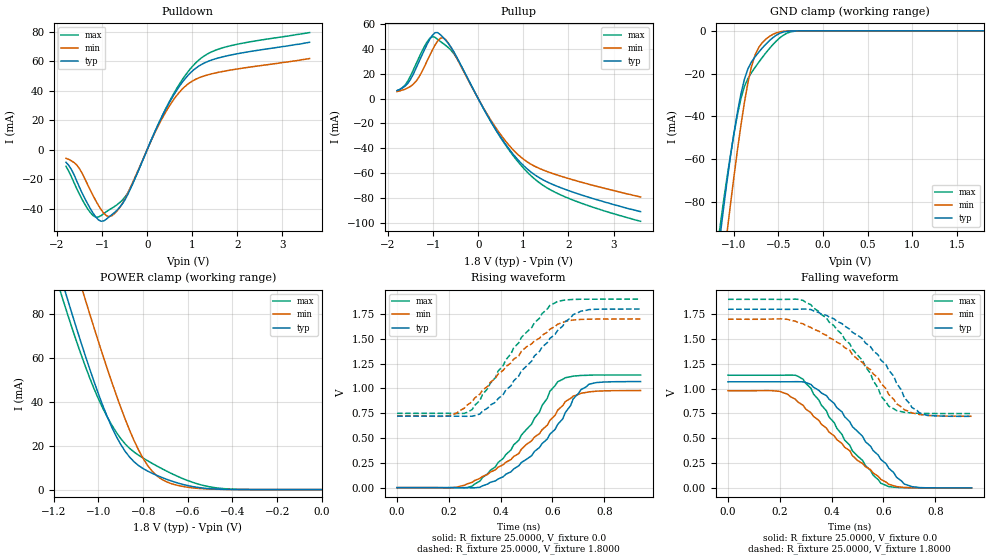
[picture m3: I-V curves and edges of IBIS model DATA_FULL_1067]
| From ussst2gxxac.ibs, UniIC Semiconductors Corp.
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|   Model DATA_FULL_1067
[Model]  DATA_FULL_1067
Model_type I/O
Polarity   Non-Inverting
Enable   Active-High
Vinl =   0.70000000V
Vinh =   1.10000000V
Vmeas =   0.90000000V
Rref =   25.00000000
Vref =   0.90000000V
C_comp   2.5240pF   2.5060pF   2.5510pF
[Temperature Range]   25.0000   95.0000   0.0
[Voltage Range]   1.8000V   1.7000V   1.9000V
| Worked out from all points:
|   slope of the pulldown table from 0 to 0.27 V, typ, clamps not added: 14.5 ohm
|   slope of the pullup table from 0 to 0.27 V, typ, clamps not added: 15.2 ohm
|   GND clamp passes 1 mA (typ) near -0.47 V on its own axis
|   POWER clamp passes 1 mA (typ) near -0.55 V on its own axis
|   rising waveform, R_fixture 25.0000, V_fixture 0.0: 20-80 % time 208ps typ, 235ps min, 197ps max; typ from 0 V to 1.07 V
|   rising waveform, R_fixture 25.0000, V_fixture 1.8000: 20-80 % time 211ps typ, 242ps min, 191ps max; typ from 0.72 V to 1.8 V
|   falling waveform, R_fixture 25.0000, V_fixture 0.0: 20-80 % time 209ps typ, 236ps min, 187ps max; typ from 1.07 V to 0 V
|   falling waveform, R_fixture 25.0000, V_fixture 1.8000: 20-80 % time 202ps typ, 233ps min, 192ps max; typ from 1.8 V to 0.72 V
[Pulldown]
|Voltage   I(typ)   I(min)   I(max)
-1.8V     -8.6mA     -5.9mA     -11.3mA
-1.56V    -21.4mA    -10.5mA    -26.6mA
-1.26V    -40mA      -27.5mA    -42.6mA
-1.14V    -45.63mA   -34.6mA    -45.75mA
-960mV    -48.21mA   -43.16mA   -43.31mA
-720mV    -42.43mA   -43.22mA   -38.43mA
-420mV    -29.74mA   -28.8mA    -28.89mA
420mV     27.8mA     25.95mA    28.32mA
720mV     43.17mA    39.09mA    44.68mA
1.02V     53.74mA    46.78mA    56.97mA
1.68V     62.9mA     52.98mA    69.04mA
3.6V      72.7mA     61.7mA     79.3mA
[Pullup]
|Voltage   I(typ)   I(min)   I(max)
-1.8V     6.5mA      5.7mA      6.3mA
-1.62V    10.1mA     7.6mA      11mA
-1.38V    24.4mA     13.9mA     27.8mA
-1.08V    47.43mA    34.44mA    48.41mA
-900mV    53.26mA    46.36mA    47.78mA
-780mV    49.42mA    49.09mA    44.52mA
-660mV    44.42mA    44.58mA    41.07mA
-420mV    29.63mA    28.82mA    29.17mA
360mV     -23.16mA   -21.82mA   -23.39mA
1.08V     -56.49mA   -50.84mA   -58.95mA
1.86V     -72.23mA   -62.83mA   -78.14mA
3.6V      -91.1mA    -79.3mA    -98.9mA
[GND_clamp]
|Voltage   I(typ)   I(min)   I(max)
-1.8V     -341.4mA   -368.9mA   -332.4mA
-1.16V    -98.84mA   -124.9mA   -94.02mA
-1.12V    -85.23mA   -110.5mA   -81.66mA
-1.08V    -72.2mA    -96.41mA   -70.06mA
-1.04V    -59.93mA   -82.62mA   -59.18mA
-920mV    -29.77mA   -44.48mA   -31.9mA
-880mV    -22.69mA   -33.57mA   -26.06mA
-800mV    -14.49mA   -16.62mA   -19.53mA
-720mV    -10.02mA   -7.817mA   -14.76mA
-560mV    -3.159mA   -1.628mA   -6.393mA
-280mV    -8.14uA    -3.578uA   -70uA
1.8V      7.234nA    32.16nA    61.22nA
[POWER_clamp]
|Voltage   I(typ)   I(min)   I(max)
-1.8V     325.1mA    352.4mA    316.2mA
-1.16V    94.14mA    121mA      86.98mA
-1.14V    87.41mA    114.1mA    80.57mA
-1.06V    61.46mA    87.09mA    56.62mA
-980mV    38.21mA    61.22mA    37.03mA
-900mV    20.56mA    37.47mA    23.27mA
-820mV    10.96mA    18mA       15.69mA
-780mV    8.467mA    11.05mA    13.18mA
-740mV    6.55mA     6.435mA    10.88mA
-640mV    2.87mA     1.791mA    5.795mA
-480mV    290.4uA    171.3uA    911.2uA
0V        7.234nA    10.13nA    70.66nA
[Ramp]
| variable   typ   min   max
dV/dt_r 0.6414/0.2041n  0.5873/0.2469n  0.6810/0.1907n
dV/dt_f 0.6478/0.1974n  0.5871/0.2419n  0.6907/0.1840n
R_load = 25.0000
[Rising Waveform]
R_fixture= 25.0000
V_fixture= 0.0
V_fixture_min= 0.0
V_fixture_max= 0.0
|time   V(typ)   V(min)   V(max)
0s        0V         0V         0V
210ps     77.35uV    -1.239mV   182.1uV
270ps     -505.2uV   37.32mV    404.8uV
380ps     68.52mV    180.7mV    210.2mV
520ps     322.6mV    472.7mV    642.2mV
590ps     538.8mV    677.2mV    971.6mV
620ps     636.9mV    780.7mV    1.067V
680ps     894.6mV    922.6mV    1.124V
740ps     1.041V     965.4mV    1.133V
940ps     1.069V     978.8mV    1.135V
[Rising Waveform]
R_fixture= 25.0000
V_fixture= 1.8000
V_fixture_min= 1.7000
V_fixture_max= 1.9000
|time   V(typ)   V(min)   V(max)
0s        720.4mV    721.5mV    748.8mV
200ps     720.4mV    724.4mV    748.8mV
290ps     720.1mV    865.5mV    786.8mV
380ps     861.2mV    1.103V     1.11V
480ps     1.177V     1.374V     1.515V
590ps     1.504V     1.597V     1.837V
620ps     1.585V     1.647V     1.878V
680ps     1.744V     1.69V      1.897V
710ps     1.779V     1.696V     1.899V
940ps     1.8V       1.7V       1.9V
[Falling Waveform]
R_fixture= 25.0000
V_fixture= 0.0
V_fixture_min= 0.0
V_fixture_max= 0.0
|time   V(typ)   V(min)   V(max)
0s        1.069V     978.8mV    1.135V
200ps     1.069V     972.1mV    1.135V
260ps     1.07V      893.5mV    1.135V
290ps     1.068V     831.6mV    1.094V
380ps     929mV      601.3mV    775.7mV
480ps     616.7mV    325.5mV    372.9mV
590ps     285.2mV    84.92mV    46.06mV
680ps     38.93mV    4.498mV    1.182mV
710ps     12.03mV    1.602mV    368.8uV
940ps     0V         0V         0V
[Falling Waveform]
R_fixture= 25.0000
V_fixture= 1.8000
V_fixture_min= 1.7000
V_fixture_max= 1.9000
|time   V(typ)   V(min)   V(max)
0s        1.8V       1.7V       1.9V
270ps     1.8V       1.667V     1.9V
320ps     1.797V     1.616V     1.845V
380ps     1.739V     1.537V     1.712V
520ps     1.502V     1.261V     1.282V
590ps     1.288V     1.054V     925.3mV
620ps     1.187V     943.4mV    823.8mV
680ps     910.4mV    788.1mV    761.1mV
740ps     752.2mV    738.4mV    750.4mV
940ps     720.5mV    721.5mV    748.8mV
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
